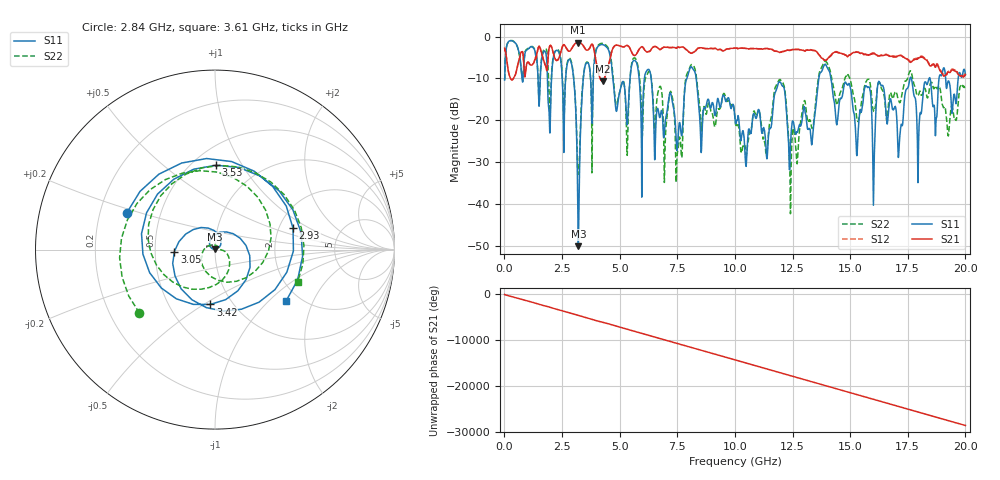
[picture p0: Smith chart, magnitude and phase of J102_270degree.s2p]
!Keysight Technologies,N5222A,MY51421036,A.10.65.16
!Date: Friday, March 31, 2023 14:55:34
!Correction: S11(Full 2 Port(1,2))
!S21(Full 2 Port(1,2))
!S12(Full 2 Port(1,2))
!S22(Full 2 Port(1,2))
!S2P File: Measurements: S11, S21, S12, S22:
# Hz S  dB  R 50
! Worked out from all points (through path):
!   2000 points, 10 MHz to 20 GHz, reference 50 ohm
!   highest |S21| = -1.46 dB at 3.2 GHz (marker M1); lowest = -10.7 dB at 4.26 GHz (marker M2)
!   group delay of S21, straight-line fit = 3.98 ns
!   lowest |S11| = -50.1 dB at 3.21 GHz (marker M3), VSWR 1.01, Z = 50 + j0.312 ohm
!   |S11| at or under -10 dB: 6.369 GHz to 7.917 GHz (1.549 GHz wide, 21.7 % of centre); 8.322 GHz to 13.64 GHz (5.318 GHz wide, 48.4 % of centre); 14.17 GHz to 17.6 GHz (3.431 GHz wide, 21.6 % of centre)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
!   |S22| runs from -42.4 to -0.9 dB; largest |S21 - S12| = 0.019
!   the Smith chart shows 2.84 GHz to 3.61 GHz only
!   S11 on the Smith chart (normalised r, x): 2.84 GHz: 0.32, +0.18; 2.93 GHz: 2.39, +0.71; 3.05 GHz: 0.63, -0.01; 3.42 GHz: 0.79, -0.53; 3.53 GHz: 0.64, +0.78; 3.61 GHz: 1.70, -1.28
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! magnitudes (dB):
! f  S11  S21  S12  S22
! 10 MHz  -10.4  -2.8  -2.7  -10.3
! 2.84 GHz  -5.5  -3.5  -3.4  -5.2
! 2.93 GHz  -6.9  -2.8  -2.8  -6.7
! 3.05 GHz  -12.9  -1.8  -1.7  -12.6
! 3.2 GHz  -47.3  -1.5  -1.4  -32.6
! 3.21 GHz  -50.1  -1.5  -1.4  -32.9
! 3.35 GHz  -16.3  -1.7  -1.7  -15.1
! 3.42 GHz  -10.3  -2.2  -2.1  -10.0
! 3.53 GHz  -6.6  -3.1  -3.0  -6.4
! 3.61 GHz  -6.2  -3.2  -3.2  -6.1
! 4.26 GHz  -1.9  -10.7  -10.6  -1.6
! 5.31 GHz  -20.6  -2.1  -2.1  -25.7
! 5.62 GHz  -5.7  -4.5  -4.4  -5.1
! 6.68 GHz  -17.7  -2.8  -2.8  -12.9
! 7.52 GHz  -25.6  -2.5  -2.5  -27.3
! 8.12 GHz  -7.3  -4.0  -4.0  -6.7
! 8.53 GHz  -26.7  -2.7  -2.6  -20.9
! 10.01 GHz  -19.8  -2.7  -2.7  -19.8
! 13.34 GHz  -25.8  -3.2  -3.2  -21.9
! 13.91 GHz  -6.6  -5.7  -5.6  -5.9
! 16.67 GHz  -17.7  -4.6  -4.5  -15.8
! 20 GHz  -9.1  -9.1  -8.8  -12.5
